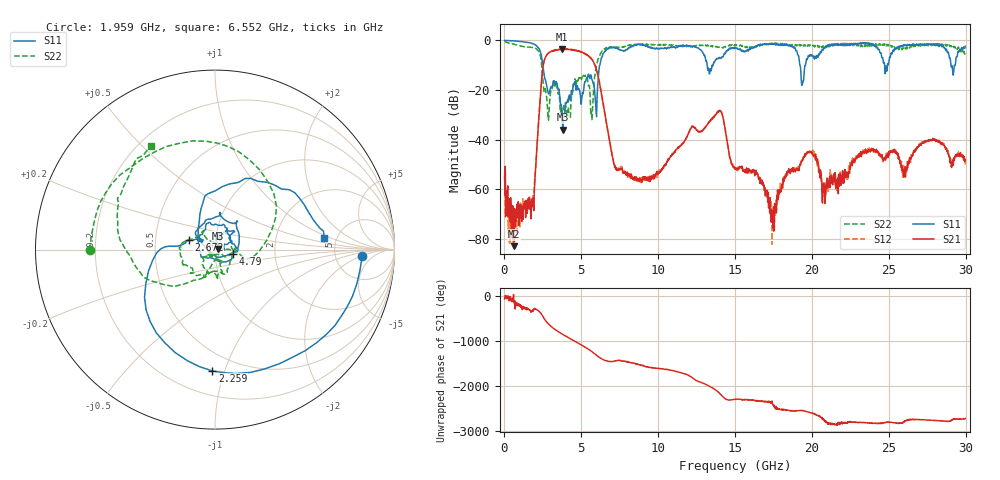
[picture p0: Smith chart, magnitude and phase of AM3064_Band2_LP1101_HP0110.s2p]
# Hz S DB R 50.0
!freq dBS11 angS11 dBS21 angS21 dBS12 angS12 dBS22 angS22
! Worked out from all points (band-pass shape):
!   1600 points, 10 MHz to 29.98 GHz, reference 50 ohm
!   highest |S21| = -3.46 dB at 3.759 GHz (marker M1); lowest = -82.9 dB at 591.1 MHz (marker M2)
!   |S21| within 3 dB of the highest: 2.693 GHz to 5.487 GHz (2.794 GHz wide, 68.3 % of centre)
!   lowest |S11| = -36.0 dB at 3.796 GHz (marker M3), VSWR 1.03, Z = 51.5 + j0.608 ohm
!   |S11| at or under -10 dB: 2.492 GHz to 6.199 GHz (3.707 GHz wide, 85.3 % of centre); 13.19 GHz to 13.56 GHz (374.5 MHz wide, 2.8 % of centre); 19.22 GHz to 19.58 GHz (357 MHz wide, 1.84 % of centre)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
!   |S22| runs from -33.1 to -0.2 dB; largest |S21 - S12| = 0.02
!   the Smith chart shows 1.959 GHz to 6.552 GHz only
!   S11 on the Smith chart (normalised r, x): 1.959 GHz: 9.68, -2.18; 2.259 GHz: 0.36, -0.91; 2.672 GHz: 0.74, +0.08; 4.79 GHz: 1.22, -0.06; 6.552 GHz: 3.97, +0.79
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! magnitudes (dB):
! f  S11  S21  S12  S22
! 10 MHz  0.0  -53.7  -54.6  -0.2
! 591.1 MHz  -0.2  -82.9  -74.0  -1.5
! 1.959 GHz  -1.7  -58.6  -56.4  -3.1
! 2.259 GHz  -3.4  -29.2  -29.2  -4.8
! 2.672 GHz  -16.1  -6.7  -6.7  -19.8
! 3.759 GHz  -30.6  -3.5  -3.5  -29.9
! 3.796 GHz  -36.0  -3.6  -3.5  -30.3
! 4.79 GHz  -19.8  -4.2  -4.2  -16.0
! 5.015 GHz  -24.1  -4.7  -4.7  -15.8
! 5.671 GHz  -15.4  -7.5  -7.4  -30.0
! 5.952 GHz  -27.5  -11.0  -11.0  -11.0
! 6.552 GHz  -4.3  -30.3  -30.3  -3.3
! 7.301 GHz  -3.2  -52.2  -52.4  -2.7
! 10 GHz  -3.4  -53.8  -53.5  -1.8
! 13.96 GHz  -6.9  -28.3  -28.5  -2.7
! 15 GHz  -2.9  -51.9  -51.5  -1.9
! 17.54 GHz  -1.6  -67.0  -68.8  -1.2
! 19.37 GHz  -17.8  -48.1  -48.1  -2.0
! 19.99 GHz  -5.8  -45.2  -45.6  -1.8
! 20.8 GHz  -2.8  -60.1  -62.8  -2.5
! 25 GHz  -8.9  -46.2  -45.5  -1.7
! 29.98 GHz  -2.4  -48.1  -50.4  -4.7
